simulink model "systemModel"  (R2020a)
settings: Solver=VariableStepAuto  StartTime=0.0  StopTime=10.0  RelTol=1e-3
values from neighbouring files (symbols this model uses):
  x0 = [0.2;0.1]    [initParams.m]

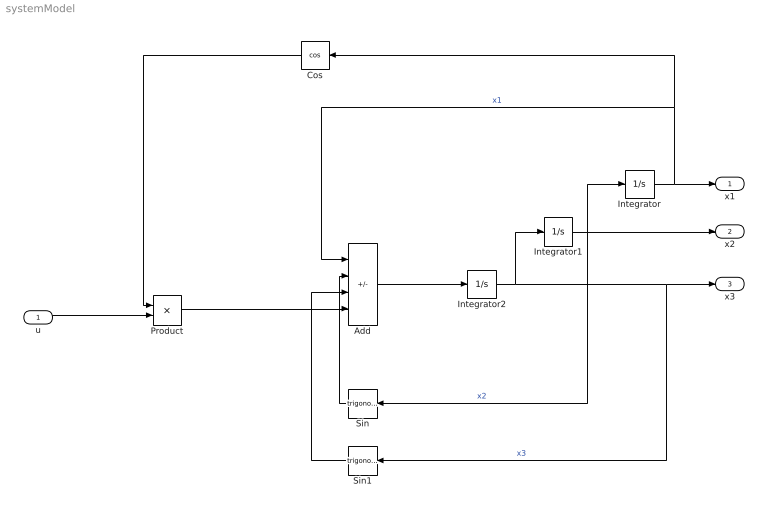
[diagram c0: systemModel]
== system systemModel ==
  u : Inport
  Add : Sum  Inputs=---+
  Cos : Trigonometry  Operator=cos
  Integrator : Integrator  InitialCondition=x0(1)
  Integrator1 : Integrator  InitialCondition=x0(2)
  Integrator2 : Integrator  InitialCondition=x0(3)
  Product : Product
  Sin : Trigonometry
  Sin1 : Trigonometry
  x1 : Outport
  x2 : Outport  Port=2
  x3 : Outport  Port=3
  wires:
  Integrator2/1 -> x3/1, Sin1/1, Integrator1/1  "x3"
  u/1 -> Product/2
  Cos/1 -> Product/1
  Sin/1 -> Add/2
  Add/1 -> Integrator2/1
  Integrator1/1 -> x2/1, Sin/1, Integrator/1  "x2"
  Product/1 -> Add/4
  Integrator/1 -> x1/1, Add/1, Cos/1  "x1"
  Sin1/1 -> Add/3
